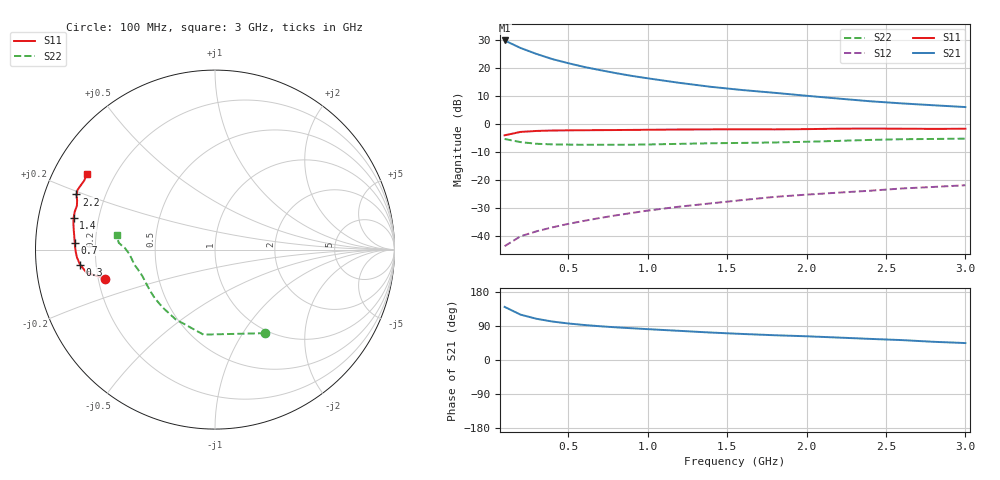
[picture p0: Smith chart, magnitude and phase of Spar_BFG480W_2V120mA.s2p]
! Filename: 2120BFG480.001
! Title: BFG480W
! Bias: Vce=2V; Ic=120mA
! Company: NXP Semiconductors NL
! User: Quality&Reliability T&D
! Measure time: 10 Nov 1999 / 11:55:25
#  MHz  S  MA  R 50
! Freq  S11  S21  S12  S22  :
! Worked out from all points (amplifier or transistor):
!   20 points, 100 MHz to 3 GHz, reference 50 ohm
!   highest |S21| = 30.0 dB at 100 MHz (marker M1)
!   |S21| within 3 dB of that: start of sweep to 214.7 MHz
!   unconditionally stable (mu >= 1): start of sweep to 103.1 MHz; 363.6 MHz to end of sweep
!   at 400 MHz: K = 1.02, MAG = 29.2 dB, |S12| = -37.0 dB
!   at 1.2 GHz: K = 1.17, MAG = 19.7 dB, |S12| = -29.5 dB
!   at 3 GHz: K = 1.16, MAG = 11.6 dB, |S12| = -21.9 dB
!   S11 on the Smith chart (normalised r, x): 100 MHz: 0.23, -0.12; 300 MHz: 0.14, -0.05; 700 MHz: 0.12, +0.02; 1.4 GHz: 0.11, +0.11; 2.2 GHz: 0.10, +0.19; 3 GHz: 0.10, +0.27
100  0.6321 -165.2  31.57 140.1  0.006541 64.6  0.5431 -59.0
200  0.7265 -169.7  23.17 119.8  0.009819 58.0  0.4779 -97.7
300  0.7567 -173.7  18.13 108.8  0.01205 58.5  0.4461 -119.5
400  0.7697 -176.6  14.65 101.5  0.0142 61.4  0.4346 -132.4
500  0.776 -179.0  12.38 96.4  0.01639 63.9  0.431 -141.1
600  0.7799 179.0  10.6 92.4  0.01857 66.0  0.4285 -147.1
700  0.7823 177.2  9.302 89.1  0.02091 67.7  0.4273 -151.7
800  0.7857 175.4  8.214 86.2  0.02328 69.3  0.4274 -155.4
900  0.7897 173.8  7.326 83.8  0.0257 70.9  0.4291 -158.6
1000  0.7942 172.2  6.634 81.4  0.02835 71.7  0.4331 -161.4
1200  0.8023 169.5  5.5 76.9  0.03335 73.0  0.4442 -165.8
1400  0.8074 167.3  4.66 72.4  0.03827 73.5  0.4555 -169.1
1600  0.8095 164.9  4.078 68.7  0.04389 74.0  0.4622 -171.9
1800  0.8073 162.4  3.643 65.3  0.04993 74.1  0.4708 -174.9
2000  0.8157 160.3  3.227 62.6  0.05476 74.4  0.4844 -178.3
2200  0.8307 158.3  2.877 59.2  0.05944 74.3  0.5026 178.9
2400  0.835 156.5  2.574 55.7  0.06433 73.6  0.5228 177.2
2600  0.8297 154.6  2.356 52.5  0.07059 72.7  0.5374 176.0
2800  0.8238 152.2  2.181 48.0  0.07522 71.2  0.544 174.2
3000  0.828 149.5  2.025 44.7  0.08062 70.3  0.5515 171.6
